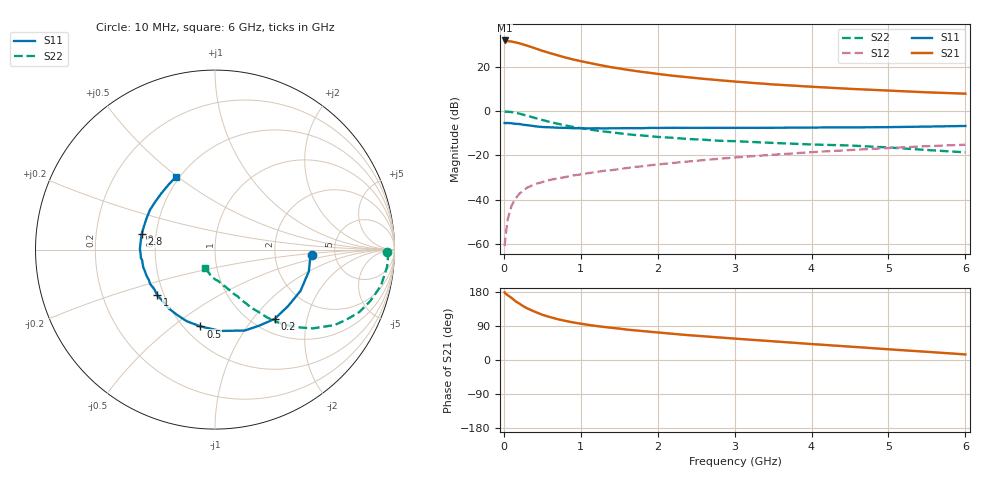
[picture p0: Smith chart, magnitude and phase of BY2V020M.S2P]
! SIEMENS Small Signal Semiconductors
! BFY420
! Si NPN RF SIEGET Grounded Emitter Transistor in MICRO-X
! VCE = 2 V  IC = 20 mA
! Common Emitter S-Parameters:  October  1996
# GHz  S  MA  R  50
!  f  S11  S21  S12  S22
! GHz  MAG  ANG  MAG  ANG  MAG  ANG  MAG  ANG
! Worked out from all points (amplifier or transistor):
!   36 points, 10 MHz to 6 GHz, reference 50 ohm
!   highest |S21| = 31.8 dB at 10 MHz (marker M1)
!   |S21| within 3 dB of that: start of sweep to 359.6 MHz
!   unconditionally stable (mu >= 1): 1.942 GHz to end of sweep
!   at 250 MHz: K = 0.30, MSG = 32.9 dB, |S12| = -35.9 dB
!   at 1.4 GHz: K = 0.92, MSG = 23.2 dB, |S12| = -26.7 dB
!   at 6 GHz: K = 1.08, MAG = 9.8 dB, |S12| = -15.2 dB
!   S11 on the Smith chart (normalised r, x): 10 MHz: 3.32, -0.26; 200 MHz: 1.24, -1.30; 500 MHz: 0.60, -0.63; 1 GHz: 0.46, -0.28; 2.8 GHz: 0.41, +0.09; 6 GHz: 0.48, +0.49
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0.01  0.5393 -3.0  38.86 178.6  0.0009 108.1  0.9586 -0.7
0.02  0.5327 -5.2  38.57 175.7  0.0014 93.1  0.9657 -1.9
0.05  0.5367 -13.0  37.59 171.0  0.0036 81.7  0.9632 -5.9
0.1  0.5291 -25.8  36.76 163.8  0.0073 80.9  0.9457 -12.4
0.15  0.5146 -37.8  35.16 155.3  0.0106 74.5  0.9122 -18.2
0.2  0.5095 -49.4  33.64 149.1  0.0135 70.9  0.8762 -23.4
0.25  0.4897 -60.1  31.64 142.3  0.0161 67.8  0.8288 -28.2
0.3  0.4804 -69.8  29.75 136.7  0.0186 66.6  0.7871 -32.3
0.4  0.4543 -86.0  26.09 127.6  0.0224 61.8  0.7005 -38.8
0.5  0.4356 -100.7  22.73 119.3  0.025 60.4  0.6269 -43.6
0.6  0.429 -111.6  20.15 113.2  0.028 57.7  0.5661 -47.4
0.7  0.4204 -120.5  17.98 107.8  0.0302 57.7  0.5166 -50.3
0.8  0.417 -129.3  16.05 103.2  0.0325 55.8  0.473 -52.7
1  0.4102 -141.6  13.27 95.8  0.0373 56.9  0.4109 -55.9
1.1  0.4038 -147.2  12.23 92.7  0.0398 56.4  0.3856 -57.7
1.6  0.4111 -165.7  8.509 80.2  0.0518 56.7  0.3005 -63.5
2.2  0.4186 179.5  6.227 69.1  0.0675 55.3  0.2488 -69.2
2.8  0.4176 168.2  4.939 59.5  0.0838 52.1  0.2135 -74.5
3.5  0.4188 156.3  3.971 49.3  0.1035 47.9  0.1909 -80.1
4.5  0.4265 141.5  3.159 35.3  0.1319 39.8  0.1669 -89.2
5.5  0.4453 125.3  2.636 21.6  0.1608 30.6  0.1322 -105.6
6  0.46 118.4  2.458 14.7  0.1739 25.7  0.1171 -117.9
